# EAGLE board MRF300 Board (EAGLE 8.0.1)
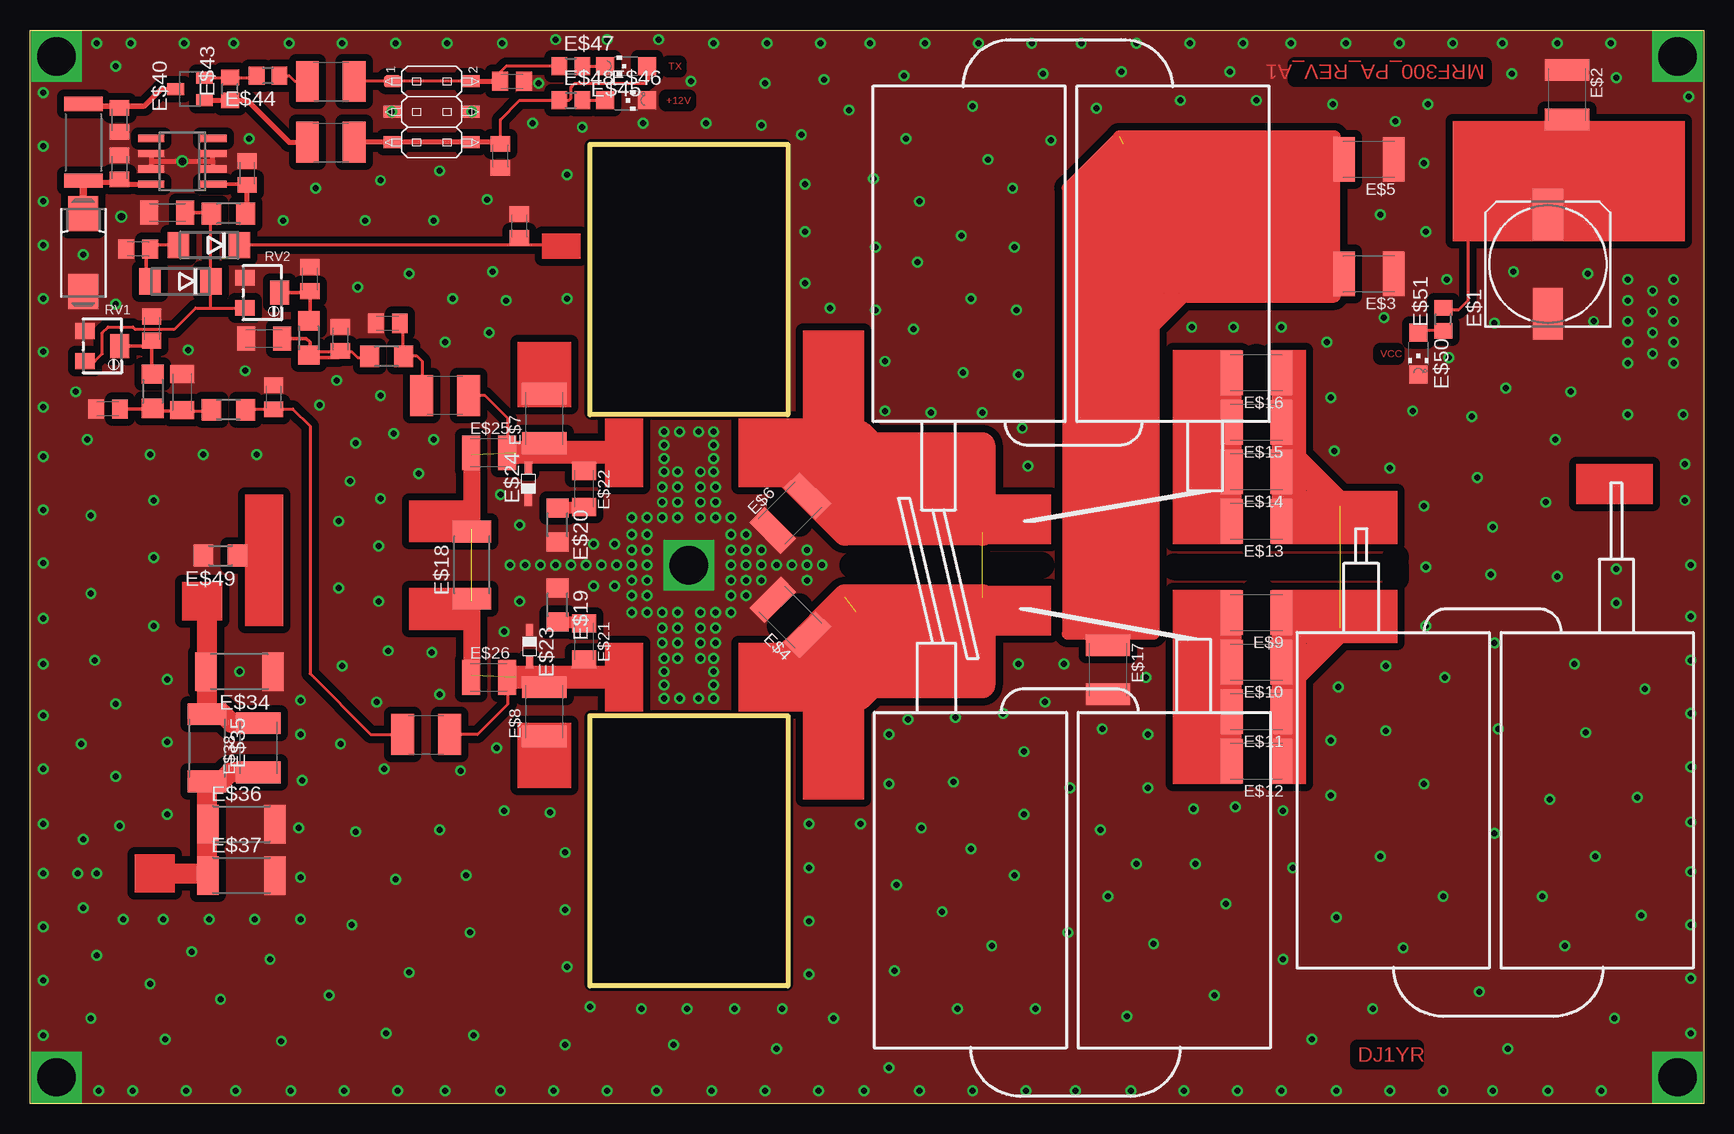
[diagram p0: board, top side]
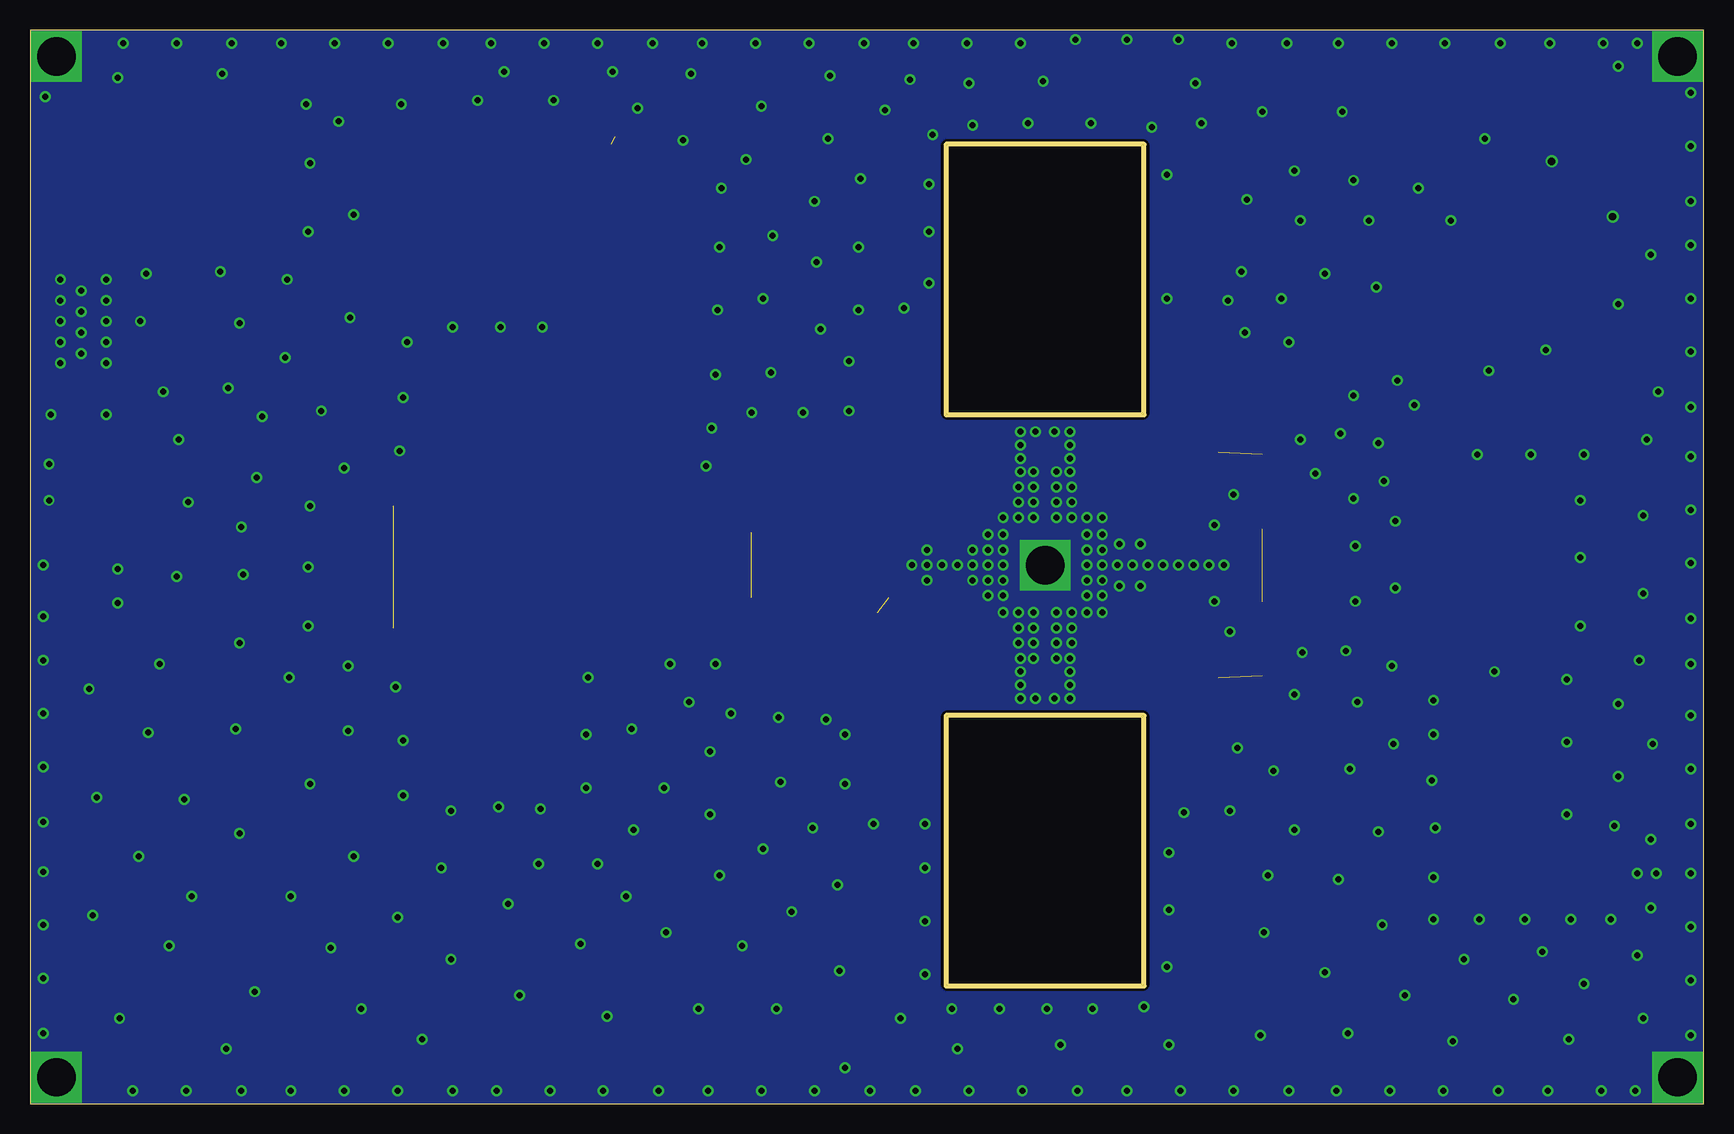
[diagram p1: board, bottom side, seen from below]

Size 139.54 x 89.53 mm. Coordinates in mm from the lower left corner, seen from the top.
Outline: 0,89.53 139.54,89.53 139.54,0 0,0 0,89.53
Copper layers (1*16): Top 0.035mm / dielectric 1.5mm / Bottom 0.035mm
Design rules "default *": minimum track width 10mil, minimum drill 24mil, track to track 8mil, track to pad 8mil, pad to pad 8mil, via to via 8mil, smd to smd 8mil, copper to edge 0mil, drill to drill 8mil, minimum pad ring 10mil, minimum via ring 8mil, stop-mask expansion 0mil, vias tented up to drill 0mil, thermal gap 10mil
tRestrict: area 46.8,57.6 to 62.9,79.9; area 46.8,10 to 63,32.2; 8 lines
bRestrict: area 46.8,10 to 63,32.2; area 46.8,57.6 to 63,79.9
Milling: 8 lines

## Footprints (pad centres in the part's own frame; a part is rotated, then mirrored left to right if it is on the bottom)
C0805K = smd 1.3 x 1.6: 1 -1,0; 2 1,0
153CLV-1014 = smd 4.3 x 2.5: + 4.15,0; - -4.15,0
C1812K = smd 1.8 x 3.7: 1 -2.05,0; 2 2.05,0
R2512 = smd 1.8 x 3.2: 1 -2.8,0; 2 2.8,0
R1206 = smd 1.6 x 1.803: 1 -1.422,0; 2 1.422,0
C1206K = smd 1.5 x 2: 1 -1.5,0; 2 1.5,0
SOD323W_INFINEON = smd 1 x 0.6: A 1.35,0; C -1.35,0
C1210K = smd 1.5 x 2.9: 1 -1.5,0; 2 1.5,0
2X3SMD = smd 1 x 1.5: 1 -2.54,-3.25; 2 -2.54,3.25; 3 0,-3.25; 4 0,3.25; 5 2.54,-3.25; 6 2.54,3.25
SC59-EBC = smd 1 x 1.4: B 0.95,-1.2; C 0,1.2; E -0.95,-1.2
R0805 = smd 1.3 x 1.5: 1 -0.95,0; 2 0.95,0
CHIPLED_1206 = smd 1.5 x 1.5: A 0,-1.75; C 0,1.75
R6332W = smd 1.2 x 3.2: 1 -3.196,0; 2 3.196,0
DO214AA = smd 1.8 x 2.2: A 2.55,0; C -2.55,0
085CS_1AR = smd 2.9 x 2.5: + 3.25,0; - -3.25,0
SO-08 = smd 0.6 x 2.2: 1 -1.905,-2.6; 2 -0.635,-2.6; 3 0.635,-2.6; 4 1.905,-2.6; 5 1.905,2.6; 6 0.635,2.6; 7 -0.635,2.6; 8 -1.905,2.6
L1812 = smd 1.9 x 3.4: 1 -1.95,0; 2 1.95,0
RTRIM5W = smd 1.3 x 1.6: 1 -1.25,-1.45; 3 1.25,-1.45 | smd 2 x 1.6: 2 0,1.45

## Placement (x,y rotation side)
100N2  100n  [C0805K]  18.1,77.6 270 top
E$1  [153CLV-1014]  126.52,70.01 90 top
E$2  [C1812K]  128.11,84.14 270 top
E$3  [C1812K]  111.6,69.22 180 top
E$4  [C1812K]  63.37,40.57 135 top
E$5  [C1812K]  111.6,78.74 180 top
E$6  [C1812K]  63.36,49.26 45 top
E$7  [C1812K]  42.86,57.15 90 top
E$8  [C1812K]  42.86,32.7 90 top
E$9  [C1812K]  102.23,40.96 180 top
E$10  [C1812K]  102.23,36.83 180 top
E$11  [C1812K]  102.23,32.7 180 top
E$12  [C1812K]  102.23,28.57 180 top
E$13  [C1812K]  102.23,48.58 180 top
E$14  [C1812K]  102.23,52.7 180 top
E$15  [C1812K]  102.23,56.83 180 top
E$16  [C1812K]  102.23,60.96 180 top
E$17  [C1812K]  89.85,36.2 270 top
E$18  [R2512]  36.83,44.93 90 top
E$19  [R1206]  43.97,41.59 270 top
E$20  [R1206]  43.97,48.26 270 top
E$21  [C1206K]  46.2,38.58 270 top
E$22  [C1206K]  46.2,51.28 270 top
E$23  [SOD323W_INFINEON]  41.64,38.15 270 top
E$24  [SOD323W_INFINEON]  41.55,51.71 90 top
E$25  [C1210K]  38.26,54.29 0 top
E$26  [C1210K]  38.26,35.56 0 top
E$27  100n  [C0805K]  10.16,64.64 90 top
E$28  470R  [R1206]  10.23,59.42 90 top
E$29  18R  [R1206]  16.55,57.87 0 top
E$30  100n  [C0805K]  6.48,57.94 180 top
E$31  100n  [C1206K]  12.71,59.35 270 top
E$32  100n  [C0805K]  20.32,58.92 90 top
E$33  100n  [C0805K]  40.79,73.21 90 top
E$34  [R2512]  17.46,36.04 180 top
E$35  [R2512]  14.76,29.69 270 top
E$36  [R2512]  17.62,23.34 0 top
E$37  [R2512]  17.62,19.05 0 top
E$38  [C1812K]  19.05,29.69 90 top
E$39  [2X3SMD]  33.5,82.71 270 top
E$40  [SC59-EBC]  13.34,84.61 90 top
E$41  100n  [C0805K]  39.22,79.03 270 top
E$42  100n  [C0805K]  40.19,85.25 0 top
E$43  [R0805]  16.67,84.61 90 top
E$44  [R0805]  19.84,85.72 180 top
E$45  [CHIPLED_1206]  49.69,86.52 90 top
E$46  [CHIPLED_1206]  49.69,83.66 270 top
E$47  [R0805]  45.09,86.52 0 top
E$48  [R0805]  45.09,83.66 0 top
E$49  [R1206]  15.88,45.72 180 top
E$50  [CHIPLED_1206]  115.73,62.55 180 top
E$51  [R0805]  117.79,65.41 90 top
E$64  100n  [C0805K]  7.47,78.08 270 top
E$65  3R9  [R6332W]  4.45,80.17 270 top
E$66  100n  [C0805K]  7.47,82.05 270 top
E$67  220R  [R1206]  16.56,74.22 0 top
E$68  100n  [C1206K]  11.45,74.3 0 top
E$69  3,9V  [DO214AA]  12.54,68.58 180 top
E$70  4148  [DO214AA]  14.92,71.6 180 top
E$71  100n  [C0805K]  9.02,71.27 180 top
E$75  100n  [C0805K]  23.33,68.76 90 top
E$76  470R  [R1206]  23.25,63.86 90 top
E$77  18R  [R1206]  29.73,62.32 0 top
E$78  100n  [C1206K]  19.5,63.81 180 top
E$79  100n  [C0805K]  25.88,63.79 270 top
E$80  100n  [C0805K]  29.82,65.08 180 top
E$83  10uF  [085CS_1AR]  4.44,70.96 90 top
IC2  78L08  [SO-08]  12.7,78.58 90 top
L1  10uH  [L1812]  33.02,30.8 0 top
L2  10uH  [L1812]  25.08,80.17 0 top
L3  10uH  [L1812]  25.08,85.25 0 top
L4  10uH  [L1812]  34.61,59.06 180 top
RV1  10K  [RTRIM5W]  6.03,63.18 270 top
RV2  10K  [RTRIM5W]  19.37,67.63 270 top

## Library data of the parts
100N2 E$1-E$22 E$25-E$38 E$41-E$44 E$47-E$49 E$51 E$64-E$68 E$71 E$75-E$80 E$83 L1-L4 RV1 RV2 = rcl
E$23 E$24 E$69 E$70 = diode
E$39 = atmel-1
E$40 = transistor
E$45 E$46 E$50 = led
IC2 = v-reg

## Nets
GND: 100N2.1 E$1.- E$2.1 E$3.1 E$4.2 E$5.1 E$6.1 E$17.2 E$19.1 E$20.2 E$23.C E$24.C E$27.2 E$30.2 E$31.1 E$32.2 E$33.2 E$34.1 E$36.2 E$37.2 E$39.3 E$39.4 E$41.2 E$42.2 E$46.C E$49.2 E$50.C E$64.1 E$66.2 E$68.1 E$71.2 E$75.2 E$78.2 E$79.1 E$80.2 E$83.- IC2.2 IC2.3 IC2.6 IC2.7 RV1.1 RV2.1

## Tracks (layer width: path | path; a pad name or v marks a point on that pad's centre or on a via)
+12V2
  Top 0.406: 9.53,83.19 4.13,83.19
D  (2 unrouted)
  Top 2.184: 66.04,37.78 66.04,38.1 68.9,40.96 77.79,40.96 77.79,36.51 69.85,36.51 67.94,38.42 76.2,38.42 76.2,39.37 69.53,39.37 69.22,39.69 | 67.31,55.88 69.22,55.88 70.17,54.93 79.38,54.93 79.38,47.62 67.94,47.62 63.5,52.07 68.26,52.07 69.53,53.34 78.11,53.34 78.11,49.53 77.79,49.21 68.26,49.21 66.99,50.48 69.22,50.48 70.48,51.75 77.15,51.75 77.15,51.12 76.83,50.8 71.12,50.8 | 63.5,37.78 67.94,42.23 79.38,42.23 79.38,34.92 70.17,34.92 69.22,33.97
G  (3 unrouted)
  Top 1.422: 36.83,54.13 36.83,47.94 | 36.83,41.91 36.83,35.72
  Top 1.93: 49.53,35.56 40.48,35.56 | 49.53,54.29 40.48,54.29
GND  (via drill 0.5, 0.6, 3.2)
  Top 0.406: 15.24,78.58 15.24,77.95 | 15.24,78.58 15.24,79.22 | 10.16,78.58 15.24,78.58 | 10.16,77.95 10.16,78.58 | 10.16,78.58 10.16,79.22
  other vias: 54.93,44.93 54.13,56.04 55.72,56.04 55.88,52.7 53.98,52.7 53.98,51.44 55.88,51.44 55.88,50.16 53.98,50.16 53.98,48.9 55.88,48.9 54.13,33.81 55.72,33.81 55.88,37.15 53.98,37.15 53.98,38.42 55.88,38.42 55.88,39.69 53.98,39.69 53.98,40.96 55.88,40.96 57.15,48.9 57.15,50.16 58.42,48.9 57.15,40.96 58.42,40.96 57.15,39.69 58.42,42.39 58.42,43.66 58.42,44.93 58.42,46.2 58.42,47.47 56.99,52.7 56.99,53.82 56.99,54.93 56.99,56.04 52.86,52.7 52.86,53.82 52.86,54.93 52.86,56.04 52.86,37.15 52.86,36.04 52.86,34.92 52.86,33.81 56.99,37.15 56.99,36.04 56.99,34.92 56.99,33.81 52.7,40.96 51.44,40.96 52.7,48.9 51.44,48.9 51.44,44.93 51.44,46.2 51.44,43.66 51.44,47.47 51.44,42.39 52.7,39.69 52.7,50.16 50.16,48.9 50.16,47.47 50.16,46.2 50.16,44.93 50.16,43.66 50.16,42.39 50.16,40.96 59.69,42.39 59.69,43.66 59.69,44.93 59.69,46.2 59.69,47.47 57.15,51.44 57.15,38.42 52.7,38.42 52.7,51.44 60.96,44.93 62.23,44.93 63.5,44.93 64.77,44.93 66.04,44.93 83.19,53.18 60.96,46.2 60.96,43.66 64.77,43.66 64.77,46.2 127.32,43.97 133.19,68.74 133.19,66.99 133.19,65.25 133.19,63.5 133.19,61.75 137,61.75 137,63.5 137,65.25 137,66.99 137,68.74 135.25,67.79 135.25,66.04 135.25,64.29 135.25,62.55 40.8,48.26 40.8,41.91 46.99,46.67 40.01,44.93 41.27,44.93 42.55,44.93 43.81,44.93 45.09,44.93 46.35,44.93 47.62,44.93 48.9,44.93 137.32,87.31 137.32,2.22 46.99,43.18 7.62,73.98 13.18,62.87 7.14,66.67 17.94,61.12 25.56,60.33 29.21,59.05 33.66,55.4 32.38,52.55 27.15,55.09 25.72,48.58 25.72,43.02 21.11,73.66 26.04,36.51 28.89,33.5 34.13,34.13 33.5,37.62 29.05,46.51 29.21,50.48 29.05,41.91 27.3,68.1 31.59,69.22 38.58,69.37 44.77,67.15 39.69,66.99 38.26,64.29 34.61,63.5 35.24,67.15 2.22,87.31 2.22,2.22 30.32,55.88 29.84,37.78 12.7,78.58 18.89,54.13 14.45,54.13 10,54.13 4.76,55.4 12.86,88.42 8.41,88.42 7.14,86.52 5.56,88.42 30.48,88.42 26.04,88.42 21.59,88.42 16.99,88.42 48.1,88.74 43.81,88.74 39.37,88.42 34.77,88.42 65.88,88.42 61.44,88.42 56.99,88.42 52.39,88.74 83.5,88.42 79.06,88.42 74.61,88.42 70.01,88.42 101.12,88.42 96.68,88.42 92.23,88.42 87.63,88.42 118.59,88.42 114.14,88.42 109.7,88.42 105.09,88.42 138.27,83.98 131.76,88.42 127.32,88.42 122.71,88.42 13.02,1.11 8.57,1.11 11.27,5.4 5.71,1.11 30.64,1.11 26.19,1.11 21.75,1.11 17.14,1.11 48.1,1.11 43.66,1.11 39.21,1.11 34.61,1.11 65.72,1.11 61.28,1.11 56.83,1.11 52.23,1.11 83.03,1.11 78.58,1.11 74.14,1.11 69.53,1.11 100.65,1.11 96.2,1.11 91.76,1.11 87.15,1.11 117.79,1.11 113.35,1.11 108.9,1.11 104.3,1.11 138.43,40.64 130.97,1.11 126.52,1.11 121.92,1.11 138.43,19.37 138.43,14.92 138.43,10.48 138.43,5.87 138.43,36.99 138.43,32.54 138.43,28.1 138.43,23.5 1.11,53.98 1.11,49.53 1.11,45.09 1.11,40.48 1.11,71.6 1.11,67.15 1.11,62.71 1.11,58.1 4.45,70.8 1.11,84.3 1.11,79.85 1.11,75.25 5.08,7.14 7.14,27.3 5.08,42.55 3.81,59.37 1.11,19.21 1.11,14.76 1.11,10.32 1.11,5.71 1.11,36.67 1.11,32.38 1.11,27.94 1.11,23.34 10.32,50.32 10.32,45.56 10.32,39.85 11.43,35.4 11.43,30.16 11.43,24.13 7.46,23.18 4.45,22.07 3.97,19.21 5.56,19.21 29.69,5.87 4.45,16.35 7.78,15.4 11.11,15.4 14.92,15.4 18.73,15.4 22.54,15.4 22.54,18.89 22.38,23.02 22.7,26.99 22.54,30.8 22.54,33.66 17.46,36.04 25.88,30 29.53,27.94 35.88,27.78 38.89,29.69 39.53,24.45 43.34,24.29 44.61,20.95 44.61,16.19 44.77,11.43 46.67,8.1 50.96,7.94 54.77,7.94 58.74,7.94 62.71,7.94 64.93,10.79 64.93,15.24 64.93,19.68 64.93,23.34 44.77,77.47 46.04,81.44 51.12,81.76 56.36,81.76 60.96,81.6 64.29,80.8 64.61,76.68 64.61,72.71 64.61,68.42 66.67,66.36 70.48,66.2 71.28,61.91 71.28,57.78 75.09,57.63 79.38,57.63 82.71,56.36 69.22,23.34 71.6,26.67 71.6,30.8 73.18,32.07 77.15,32.23 81.12,32.54 82.39,36.67 86.2,36.67 93.03,35.56 84.61,33.5 89.38,31.27 93.19,30.8 93.19,26.35 97,24.61 100.49,24.77 104.46,24.45 108.43,25.72 108.43,30.32 109.06,34.77 113.03,36.51 116.36,39.85 116.36,44.77 116.2,49.85 113.35,53.02 108.74,54.45 108.43,58.9 108.11,63.5 104.3,64.77 100.33,64.77 96.84,64.77 70.48,71.44 70.33,77.15 68.26,82.87 61.28,85.09 55.09,85.25 121.92,48.1 36.83,82.71 82.39,60.8 82.23,66.2 82.07,71.44 81.92,76.36 85.09,80.33 88.9,83.03 95.89,83.66 102.23,83.66 108.58,83.34 112.55,74.14 112.87,65.56 113.82,81.92 118.11,68.74 122.08,65.09 123.03,59.69 128.43,59.37 133.19,57.47 127.16,55.4 126.36,50.16 121.76,44.13 120.65,52.23 115.25,57.78 118.27,62.23 122.08,38.42 128.75,36.67 132.24,44.61 132.24,41.75 134.62,34.61 117.95,35.56 113.03,31.11 122.4,31.27 129.7,30.96 133.99,25.56 126.68,25.4 116.2,26.67 112.55,20.64 122.08,22.54 130.49,20.64 134.3,15.72 126.05,17.3 117.79,17.3 108.9,15.56 111.92,7.94 114.46,13.02 120.81,9.37 127.95,13.18 132.08,7.14 123.19,4.6 106.84,5.4 105.25,19.68 104.46,12.06 99.69,16.67 92.23,20 86.68,26.35 76.99,26.83 78.42,21.27 72.23,18.26 89.85,17.3 93.66,13.34 98.74,9.05 91.44,7.3 82.87,24.13 97.16,20 89.22,22.86 82.87,29.37 74.3,23.02 76.04,16.03 82.07,19.05 80.17,13.18 72.07,11.11 77.31,7.94 83.82,7.94 86.52,14.29 66.99,7.14 71.6,3.02 62.23,4.6 53.66,4.92 44.61,4.92 36.99,5.71 36.67,14.29 34.13,22.86 27.15,22.7 26.83,14.92 24.92,9.05 15.88,8.73 10,10 31.59,10.95 30.48,18.73 5.56,12.38 4.29,30 7.14,33.34 5.4,36.99 5.08,49.05 73.66,64.61 77.79,60.96 78.42,67.15 73.98,70.17 74.14,75.25 77.63,72.39 79.85,78.74 73.03,80.49 66.2,85.41 72.87,85.72 78.58,83.19 84.45,85.88 90.96,86.04 100.01,86.04 116.52,83.34 120.17,57.31 123.51,85.88 132.24,85.57 123.67,69.37 130.33,65.25 129.86,69.22 116.2,78.42 116.36,72.71 137.95,53.34 137.95,50.32 137.79,57.47 138.43,44.93 30.16,82.71 18.26,80.49 23.81,76.36 27.94,73.66 29.21,76.99 34.13,77.79 33.66,73.66 38.1,75.41 41.91,81.76 20.95,5.24 20,12.06 13.49,12.7 36.35,19.05 26.67,51.91 48.74,46.67 48.74,43.18 42.39,85.09 24.13,58.26 39.53,39.37 39.21,50.8
  pour Top (isolate 0.61, no thermals): 0,89.53 139.54,89.53 139.54,0 0,0
  pour Bottom (isolate 0.61): 0,89.53 139.54,89.53 139.54,0 0,0
S$1
  Top 0.254: 44.29,86.52 39.69,86.52 39.21,86.04 39.21,85.25 | 36.67,85.25 26.99,85.25
  Top 0.406: 36.67,85.25 39.21,85.25
S$2
  Top 0.254: 46.04,86.52 47.94,86.52
S$3
  Top 2.184: 63.18,36.51 63.5,36.51 63.82,36.83
S$4
  Top 0.254: 46.04,83.66 47.94,83.66
S$5  (1 unrouted)
  Top 2.184: 105.09,33.34 105.09,35.56 109.22,39.69 | 109.22,49.85 105.09,53.98
S$6
  Top 0.254: 39.85,35.56 39.85,33.34 37.31,30.8 35.08,30.8
S$7
  Top 0.254: 117.79,64.45 115.73,64.45
S$8
  Top 0.254: 119.86,72.39 119.86,66.99 119.06,66.2 117.63,66.2
S$9
  Top 1.016: 44.13,40.16 46.2,40.16
S$10
  Top 1.016: 46.2,49.69 44.29,49.69
S$11
  Top 0.254: 15.08,66.36 15.08,74.3
  Top 0.305: 15.08,74.3 13.18,74.3
  Top 0.406: 15.08,74.3 15.24,74.3
S$12
  Top 0.305: 7.46,63.18 9.84,63.18
S$13
  Top 1.676: 14.76,32.7 14.76,42.07
S$14
  Top 0.254: 17.62,57.94 21.91,57.94 23.34,56.52 23.34,35.88 28.42,30.8 31.27,30.8
S$15
  Top 0.305: 15.24,76.68 18.26,76.68
S$16
  Top 0.305: 10.16,61.12 10.16,63.18
  Top 0.406: 10.16,63.18 9.84,63.34
S$17
  Top 0.254: 10,57.78 14.92,57.78
  Top 0.305: 10,57.78 12.38,57.78
S$18
  Top 0.305: 10,57.94 7.62,57.94
S$19
  Top 0.254: 39.85,54.13 39.85,57.15 37.94,59.05 36.67,59.05
S$20
  Top 0.61: 4.45,74.14 4.45,76.68
S$21
  Top 0.254: 23.18,62.71 26.83,62.71 27.3,62.23 28.42,62.23
S$22
  Top 0.254: 31.11,62.23 31.11,65.09
S$23
  Top 0.254: 31.27,62.39 32.23,62.39 32.7,61.91 32.7,59.05 32.86,59.05
S$25
  Top 1.676: 14.76,18.89 14.76,26.83
S$26
  Top 0.254: 12.7,71.6 10,71.6
S$27
  Top 0.254: 4.29,61.91 5.4,61.91 6.03,62.55 6.03,64.29 6.51,64.77 8.57,64.77 8.73,64.61 12.06,64.61 13.81,66.36 17.78,66.36
  Top 0.305: 4.29,61.91 4.45,61.91
S$28
  Top 1.676: 19.21,31.75 16.83,31.75 16.03,32.54
S$29
  Top 1.676: 19.05,27.62 16.67,27.62 15.88,26.83
S$30
  Top 0.406: 5.08,83.19 9.53,83.19 10.95,84.61 12.06,84.61
S$31
  Top 1.676: 10.64,19.21 14.45,19.21
S$32
  Top 0.406: 14.61,83.66 18.1,83.66 21.59,80.17 23.18,80.17
S$33
  Top 0.254: 39.21,80.17 39.21,82.07 40.8,83.66 44.93,83.66 45.09,83.82 45.09,84.77 45.4,85.09 51.28,85.09 51.59,85.41 51.59,86.36
  Top 0.406: 26.99,80.17 39.21,80.17 39.37,80.17 39.53,80.33
S$35
  Top 0.254: 14.61,85.57 18.89,85.57
S$36
  Top 0.254: 20.64,85.72 21.59,85.72 22.07,85.25 23.5,85.25
S$60
  Top 0.406: 7.3,76.68 10,76.68
S$62
  Top 0.406: 4.13,76.83 7.14,76.83
S$63
  Top 0.406: 18.1,74.61 18.1,76.52
S$65
  Top 0.305: 9.68,71.75 9.68,68.58
S$69
  Top 0.305: 20.8,67.63 23.18,67.63
S$70
  Top 0.305: 23.34,65.56 23.34,67.63
  Top 0.406: 23.34,67.63 23.18,67.79
S$71
  Top 0.305: 23.34,62.23 25.72,62.23
S$72
  Top 0.305: 21.11,63.82 23.02,63.82 23.34,63.5 23.34,62.55
TEMPSENS
  Top 0.254: 44.61,71.6 17.46,71.6
VCC  (1 unrouted)
  Top 1.016: 87.31,68.42 87.31,76.2 91.12,80.01 107.95,80.01 107.95,68.1 93.98,68.1 93.98,66.83 94.46,66.36 94.46,66.83 95.25,67.63 | 86.68,65.09 86.68,39.21 93.66,39.21 93.66,64.77 96.2,67.31 108.74,67.31 108.74,80.64 90.81,80.64 86.52,76.36 86.52,39.21
(copper drawn outside any net)
  shapes: Top area x30

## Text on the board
Top: MRF300_PA_REV_A1 | TX | +12V | VCC | DJ1YR
tValues: BC517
